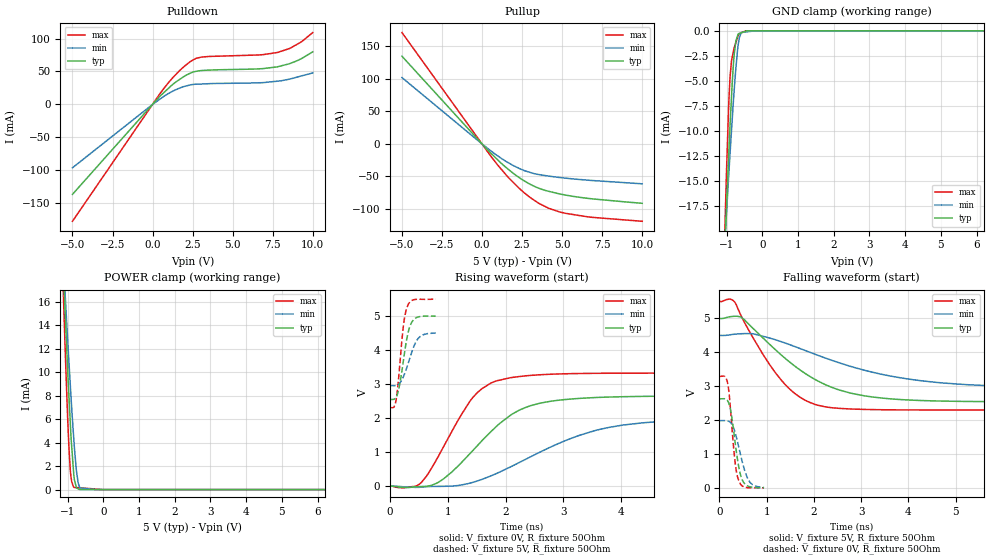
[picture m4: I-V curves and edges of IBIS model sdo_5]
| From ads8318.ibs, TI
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|   sdo_5 Model
[Model]   sdo_5
Model_type   3-state
Polarity   Inverting
Enable   Active-High
Vmeas = 2.5
Vref = 2.5
Cref = 5pF
Rref = 50
|   typ   min   max
|   (Nom PVT)   (Fast PVT)   (Slow PVT)
|C_comp from frequency method
|Average
|C_comp   2.549e-12   2.191e-12   3.191e-12
|ON state : BUFFER OUTPUT TURNED HIGH
|C_comp   2.549e-12   2.191e-12   3.191e-12
|OFF state: BUFFER IN HIGH IMPEDANCE
|C_comp   1.170e-12   9.925e-13   1.358e-12
|C_comp from LC tank method
C_comp   1.087e-12   9.649e-13   1.276e-12
| Where nom  PVT is Nominal Process,  5V,  28C
|   Fast PVT is Strong Process,   5.5V,  -40C
|   Slow PVT is Weak Process,   4.5V,  89C
[Voltage Range]   5   4.5   5.5
|Ambient Temperature   25   85   -40
|Junction Temperature
[Temperature Range]   28   89   -40
[Pullup Reference]   5   4.5   5.5
[Pulldown Reference]   0   0   0
[Power Clamp Reference]   5   4.5   5.5
[GND Clamp Reference]   0   0   0
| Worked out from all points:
|   slope of the pulldown table from 0 to 0.75 V, typ, clamps not added: 39.6 ohm
|   slope of the pullup table from 0 to 0.75 V, typ, clamps not added: 39.4 ohm
|   GND clamp passes 1 mA (typ) near -0.74 V on its own axis
|   POWER clamp passes 1 mA (typ) near -0.82 V on its own axis
|   falling waveform, V_fixture 5V, R_fixture 50Ohm: 20-80 % time 1.41ns typ, 2.17ns min, 932ps max; typ from 5 V to 2.54 V
|   rising waveform, V_fixture 0V, R_fixture 50Ohm: 20-80 % time 977ps typ, 1.58ns min, 695ps max; typ from 0 V to 2.64 V
|   rising waveform, V_fixture 5V, R_fixture 50Ohm: 20-80 % time 140ps typ, 191ps min, 107ps max; typ from 2.54 V to 4.98 V
|   falling waveform, V_fixture 0V, R_fixture 50Ohm: 20-80 % time 162ps typ, 220ps min, 125ps max; typ from 2.63 V to 0.007 V
[Pulldown]
|   Voltage   I(typ)   I(min)   I(max)
-5V       -136.5mA   -96.2mA    -177.4mA
4.5mV     122.8uA    86.55uA    166.3uA
599.5mV   15.53mA    10.4mA     20.84mA
1.243V    29.95mA    19.82mA    40.04mA
2.035V    43.43mA    27.56mA    58.91mA
2.712V    50.17mA    30.61mA    69.89mA
3.08V     51.44mA    30.99mA    71.91mA
6.6V      53.91mA    32.79mA    75.02mA
7.799V    57.06mA    35.24mA    78.77mA
8.575V    61.99mA    38.51mA    85.05mA
9.295V    69.45mA    43.2mA     94.94mA
10V       79.81mA    47.78mA    109mA
[GND Clamp]
|   Voltage   I(typ)   I(min)   I(max)
-5V       -400.3mA   -284.6mA   -619.9mA
-1.089V   -25.13mA   -23.49mA   -25.18mA
-1.026V   -19.72mA   -19.59mA   -17.04mA
-935mV    -11.91mA   -14.1mA    -6.919mA
-902mV    -9.355mA   -12.16mA   -4.572mA
-863.5mV  -6.68mA    -10.01mA   -3.035mA
-785mV    -2.283mA   -5.804mA   -1.678mA
-740mV    -1.021mA   -3.727mA   -1.168mA
-670.5mV  -292.4uA   -1.271mA   -459.4uA
-589.5mV  -190.7uA   -169.4uA   -200.6uA
-462mV    -34.14uA   -113.6uA   -2.218uA
10V       0A         0A         0A
[Pullup]
|   Voltage   I(typ)   I(min)   I(max)
-5V       135mA      102.1mA    171.4mA
610.5mV   -15.7mA    -11.77mA   -20.81mA
1.672V    -39.63mA   -29.33mA   -52.36mA
2.673V    -57.37mA   -41.32mA   -75.98mA
3.509V    -67.79mA   -46.93mA   -90.79mA
4.147V    -72.78mA   -49.4mA    -98.86mA
5.192V    -78.52mA   -52.54mA   -106.7mA
6.88V     -84.49mA   -56.26mA   -112.9mA
10V       -91.33mA   -61.33mA   -119mA
[POWER Clamp]
|   Voltage   I(typ)   I(min)   I(max)
-5V       182.4mA    165mA      207.6mA
-1.116V   18.5mA     19.21mA    16.42mA
-1.111V   18.19mA    18.96mA    16mA
-1.056V   14.26mA    15.91mA    10.9mA
-990mV    9.591mA    12.29mA    5.471mA
-957mV    7.631mA    10.59mA    3.268mA
-924mV    5.672mA    8.896mA    1.665mA
-885.5mV  3.686mA    6.957mA    682.5uA
-810mV    832.5uA    3.584mA    186.2uA
-751.5mV  160.8uA    1.575mA    172.8uA
-670mV    11.58uA    238uA      154uA
10V       0A         0A         0A
[Ramp]
R_load = 50
|   typ   min   max
dV/dt_r   1.58653/9.76071e-10   1.19646/1.59606e-09   1.98763/6.93369e-10
dV/dt_f   1.47563/1.40837e-09   0.932423/2.24155e-09   1.91957/9.31192e-10
[Falling Waveform]
V_fixture = 5V
V_fixture_min = 4.5V
V_fixture_max = 5.5V
R_fixture = 50Ohm
|   Time   V(typ)   V(min)   V(max)
0s        5V         4.5V       5.5V
300ps     5.063V     4.533V     5.517V
520ps     4.973V     4.553V     4.91V
1.2ns     4.059V     4.366V     3.372V
1.625ns   3.564V     4.156V     2.757V
2.03ns    3.196V     3.942V     2.463V
2.745ns   2.81V      3.6V       2.334V
3.45ns    2.651V     3.349V     2.309V
4.745ns   2.563V     3.096V     2.301V
7.085ns   2.542V     2.97V      2.301V
[Rising Waveform]
V_fixture = 0V
V_fixture_min = 0V
V_fixture_max = 0V
R_fixture = 50Ohm
|   Time   V(typ)   V(min)   V(max)
0s        1.456nV    1.632nV    1.35nV
235ps     -38.36mV   -18.81mV   -49.74mV
540ps     -10.89mV   -29.78mV   104.8mV
925ps     211.5mV    -5.143mV   1.151V
1.395ns   975.6mV    93.88mV    2.519V
1.855ns   1.775V     381mV      3.092V
2.245ns   2.236V     700.9mV    3.215V
2.59ns    2.431V     994.4mV    3.265V
3.775ns   2.612V     1.719V     3.31V
6.49ns    2.644V     1.979V     3.314V
[Rising Waveform]
V_fixture = 5V
V_fixture_min = 4.5V
V_fixture_max = 5.5V
R_fixture = 50Ohm
|   Time   V(typ)   V(min)   V(max)
0s        2.541V     2.946V     2.301V
69.04ps   2.546V     2.946V     2.319V
107.9ps   2.609V     2.951V     2.539V
158ps     2.889V     3.001V     3.32V
232ps     3.675V     3.207V     4.693V
267.8ps   4.083V     3.36V      5.071V
305.5ps   4.436V     3.548V     5.286V
381ps     4.815V     3.948V     5.446V
494.2ps   4.962V     4.341V     5.478V
792.5ps   4.982V     4.49V      5.482V
[Falling Waveform]
V_fixture = 0V
V_fixture_min = 0V
V_fixture_max = 0V
R_fixture = 50Ohm
|   Time   V(typ)   V(min)   V(max)
0s        2.63V      1.988V     3.291V
116.4ps   2.632V     1.989V     3.286V
172.7ps   2.574V     1.981V     3.098V
208.5ps   2.459V     1.96V      2.733V
241.1ps   2.266V     1.921V     2.201V
340.7ps   1.253V     1.591V     650.8mV
415.6ps   571.8mV    1.168V     193mV
489.8ps   219.9mV    737.5mV    53.39mV
620.9ps   47.33mV    221.8mV    9.765mV
943.8ps   6.934mV    16.85mV    5.582mV
